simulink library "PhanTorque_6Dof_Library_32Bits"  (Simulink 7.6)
settings: Solver=ode45  StartTime=0.0  StopTime=10.0  RelTol=1e-3
undefined symbols (not defined in the file or in its folder): Phantom_Jacobian, Phantom_Jacobian_Trans

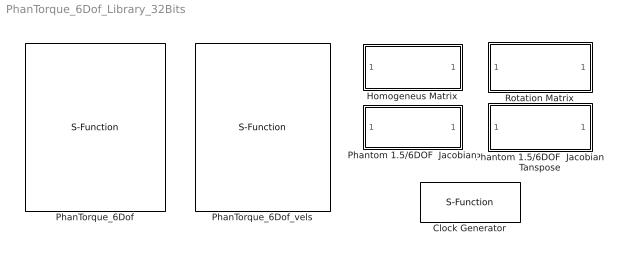
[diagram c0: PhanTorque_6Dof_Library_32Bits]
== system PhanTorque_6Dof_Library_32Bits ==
  Clock Generator : S-Function  FunctionName=PHANToM_RealTime  EnableBusSupport=off
  Homogeneus Matrix : Subsystem
  PhanTorque_6Dof : S-Function  FunctionName=PhanTorque_6Dof  Parameters=Haptic_Name  EnableBusSupport=off  mask{Haptic_Name='Default PHANToM'}
      mask prompts: Haptic_Name "Haptic Name"
      mask help: Input: tau--> Control Torques (3x1) Outputs: q-->Joints Position (3x1) p-->Cartesian Position (x,y,z, 3x1) h-->Homogeneus Transformation Matrix (vector form, 16x1) S-Function Parameter: Haptic Name--> Name as appear on the "PHANToM Test" program
  PhanTorque_6Dof_vels : S-Function  FunctionName=PhanTorque_6Dof_damp_vels  Parameters=Haptic_Name,kd  EnableBusSupport=off  mask{Haptic_Name='Default PHANToM', kd=0}
      mask prompts: Haptic_Name "Haptic Name"; kd "kd Gain"
      mask help: Input: tau--> Control Torques (3x1) Outputs: q-->Joints Position (3x1) p-->Cartesian Position (x,y,z, 3x1) v-->Linear Velocity (vx,vy,vz, 3x1) w-->Angular Velocity (wx,wy,wz, 3x1) h-->Homogeneus Transformation Matrix (vector form, 16x1) S-Function Parameter: Haptic Name--> Name as appear on the "PHANToM Test" program. Ex:'Default PHANToM' kd Gain--> Gain for internal damping. It affects only to the first 3 joints (q1,q2,q3), kd Gain=0 dissable this feature. Recommended test value <.001.
  Phantom 1.5/6DOF  Jacobian : Subsystem
  Phantom 1.5/6DOF  Jacobian Tanspose : Subsystem
  Rotation Matrix : Subsystem

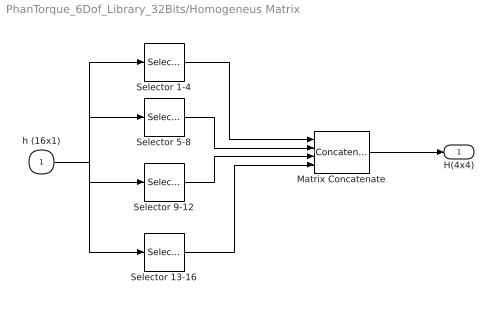
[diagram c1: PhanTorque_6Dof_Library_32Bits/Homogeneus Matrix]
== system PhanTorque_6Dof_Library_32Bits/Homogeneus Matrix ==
  h (16x1) : Inport  PortDimensions=16
  Matrix Concatenate : Concatenate  NumInputs=4  Mode=Multidimensional array  ConcatenateDimension=2
  Selector 1-4 : Selector  InputPortWidth=16  IndexOptions=Index vector (dialog)  Indices=[1 2 3 4]  OutputSizes=1
  Selector 13-16 : Selector  InputPortWidth=16  IndexOptions=Index vector (dialog)  Indices=[13 14 15 16]  OutputSizes=1
  Selector 5-8 : Selector  InputPortWidth=16  IndexOptions=Index vector (dialog)  Indices=[5 6 7 8]  OutputSizes=1
  Selector 9-12 : Selector  InputPortWidth=16  IndexOptions=Index vector (dialog)  Indices=[9 10 11 12]  OutputSizes=1
  H(4x4) : Outport  PortDimensions=[4 4]
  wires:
  h (16x1)/1 -> Selector 13-16/1, Selector 9-12/1, Selector 5-8/1, Selector 1-4/1
  Matrix Concatenate/1 -> H(4x4)/1
  Selector 13-16/1 -> Matrix Concatenate/4
  Selector 9-12/1 -> Matrix Concatenate/3
  Selector 5-8/1 -> Matrix Concatenate/2
  Selector 1-4/1 -> Matrix Concatenate/1

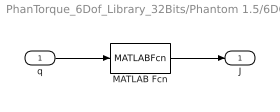
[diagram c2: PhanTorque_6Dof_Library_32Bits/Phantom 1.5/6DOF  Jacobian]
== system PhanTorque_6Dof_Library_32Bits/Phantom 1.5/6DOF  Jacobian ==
  q : Inport  PortDimensions=6
  MATLAB Fcn : MATLABFcn  MATLABFcn=Phantom_Jacobian(u)  OutputDimensions=[6 6]  Output1D=off
  J : Outport  PortDimensions=[6 6]
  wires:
  q/1 -> MATLAB Fcn/1
  MATLAB Fcn/1 -> J/1

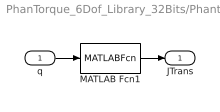
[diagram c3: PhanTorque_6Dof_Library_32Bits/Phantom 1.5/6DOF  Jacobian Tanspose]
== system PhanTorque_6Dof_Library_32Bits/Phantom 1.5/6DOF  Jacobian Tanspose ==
  q : Inport  PortDimensions=6
  MATLAB Fcn1 : MATLABFcn  MATLABFcn=Phantom_Jacobian_Trans(u)  OutputDimensions=[6 6]  Output1D=off
  JTrans : Outport  PortDimensions=[6 6]
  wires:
  q/1 -> MATLAB Fcn1/1
  MATLAB Fcn1/1 -> JTrans/1

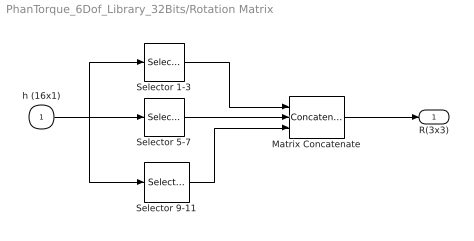
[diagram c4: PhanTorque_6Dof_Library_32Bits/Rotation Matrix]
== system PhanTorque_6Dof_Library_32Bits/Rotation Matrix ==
  h (16x1) : Inport  PortDimensions=16
  Matrix Concatenate : Concatenate  NumInputs=3  Mode=Multidimensional array  ConcatenateDimension=2
  Selector 1-3 : Selector  InputPortWidth=16  IndexOptions=Index vector (dialog)  Indices=[1 2 3]  OutputSizes=1
  Selector 5-7 : Selector  InputPortWidth=16  IndexOptions=Index vector (dialog)  Indices=[5 6 7]  OutputSizes=1
  Selector 9-11 : Selector  InputPortWidth=16  IndexOptions=Index vector (dialog)  Indices=[9 10 11]  OutputSizes=1
  R(3x3) : Outport  PortDimensions=[3 3]
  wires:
  h (16x1)/1 -> Selector 9-11/1, Selector 1-3/1, Selector 5-7/1
  Matrix Concatenate/1 -> R(3x3)/1
  Selector 9-11/1 -> Matrix Concatenate/3
  Selector 5-7/1 -> Matrix Concatenate/2
  Selector 1-3/1 -> Matrix Concatenate/1
